FUNCTION_BLOCK FB83
TITLE =Halt Velocity Movement
//*****************************************************************************
//* maxon motor ag
//* R&D
//* all rights reserved
//*****************************************************************************
//* Summary:  Halt with position profile set by SetVelocityProfile
//*
//* Remarks:
//*
//* Created under: STEP7 REV5.2+SP1
//*****************************************************************************
//* History:
//* 18.05.2004 | INA   first release
//*
//*
//*****************************************************************************
//

AUTHOR:INA
FAMILY:ProVeloM
NAME:HaltVelo
VERSION:00.01


VAR_INPUT

Write : BOOL //A rising edge start the command

  NodeID : BYTE //Adress of the maxon device

END_VAR
VAR_OUTPUT
  Done : BOOL //Data valid flag is TRUE if data were available

  Err : BOOL //Error flag is TRUE if an Error has occured, see ErrNo for more details

  ErrNo : DINT //Contains detailed error information

END_VAR
VAR
  xEdgeMerker : BOOL //Edge Merker

  xEdgeFlag : BOOL //Edge Flag

  xStep : INT
  xStopProfile : WORD  := W#16#10F
END_VAR

BEGIN

NETWORK
TITLE = Activate the service function
//

// SDO Write "Halt Velocity Movement"

       U    #Write
       FP   #xEdgeFlag                   // recognize a positiv edge of the Read signal
       =    #xEdgeMerker                 // and set the xEdgeMerker for one cycle to true

       L    #xStep
       L    0
       ==I
       U    #xEdgeMerker
       SPB  nstp                         // iStep = 1 -> fnc1

       L    #xStep                       // jump list
       SPL  List
       SPA  rdef
       SPA  fnc1
       SPA  fncE
List  :SPA  rdef

rdef  :NOP  0
       R    #Done                        // reset Done
       R    #Err
       L    0
       T    #xStep                       // iStep = 0
       SPA  end

fnc1  :NOP  0
       CALL FC15
         NodeID:=#NodeID
         Index:=DW#16#00006040
         SubIndex:=DW#16#00000000
         ValueIn:=#xStopProfile
         RET_VAL:=#Done
         Err:=#Err
         ErrNo:=#ErrNo

fncE  :NOP  0
       L    0
       T    #xStep
       SPA  end

nstp  :NOP  0
       L    #xStep
       INC            1
       T    #xStep

end   :NOP  0
END_FUNCTION_BLOCK
